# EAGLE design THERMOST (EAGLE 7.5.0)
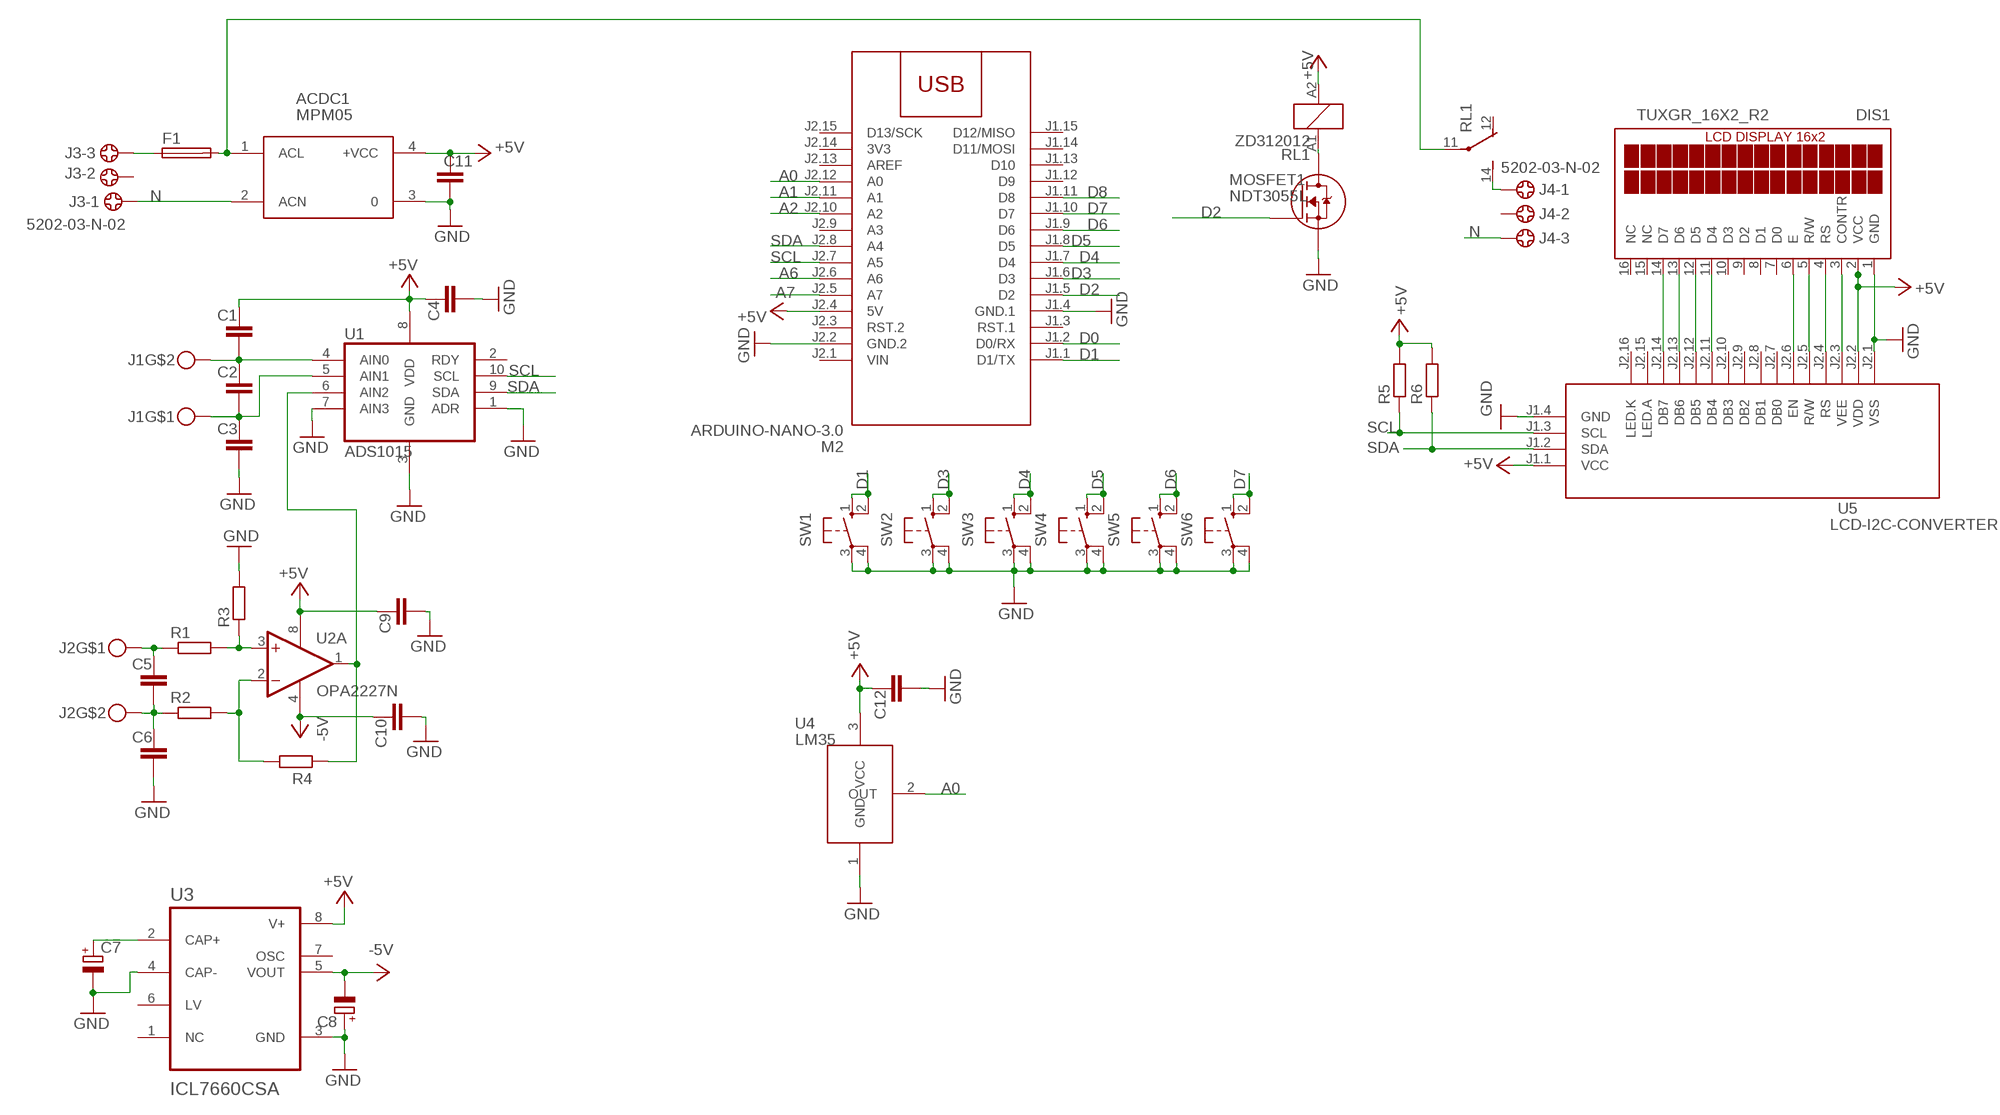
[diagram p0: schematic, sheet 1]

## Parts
ACDC1  MPM05  [MPM05]
C1  C-EUC1206  [C1206]
C2  C-EUC1206  [C1206]
C3  C-EUC1206  [C1206]
C4  C-EUC1206  [C1206]
C5  C-EUC1206  [C1206]
C6  C-EUC1206  [C1206]
C7  CPOL-EUSMCB  [SMC_B]
C8  CPOL-EUSMCB  [SMC_B]
C9  C-EUC1206  [C1206]
C10  C-EUC1206  [C1206]
C11  C-EUC1206  [C1206]
C12  C-EUC1206  [C1206]
DIS1  TUXGR_16X2_R2  [TUXGR_16X2_R2]
F1  FUSEBLANK_5X20MM  [FUSE_HOLDER_5X20MM]
J1  MKDSN1,5-2-5,08  [MKDSN1,5-2-5,08]
J2  MKDSN1,5-2-5,08  [MKDSN1,5-2-5,08]
J3  5202-03-N-02  [5202-03-N-02]
J4  5202-03-N-02  [5202-03-N-02]
M2  ARDUINO-NANO-3.0  [ARDUINO-NANO-3.0]
MOSFET1  NDT3055L  [SOT223-4]
R1  R-EU_R1206  [R1206]
R2  R-EU_R1206  [R1206]
R3  R-EU_R1206  [R1206]
R4  R-EU_R1206  [R1206]
R5  R-EU_R1206  [R1206]
R6  R-EU_R1206  [R1206]
RL1  ZD312012  [ZD1]
SW1  40-XX  [B3F-40XX]
SW2  40-XX  [B3F-40XX]
SW3  40-XX  [B3F-40XX]
SW4  40-XX  [B3F-40XX]
SW5  40-XX  [B3F-40XX]
SW6  40-XX  [B3F-40XX]
U1  ADS1015  [ADS1015]
U2  OPA2227N  [DIL08]
U3  ICL7660CSA  [SOIC127P600X175-8N]
U4  LM35  [TO92]
U5  LCD-I2C-CONVERTER  [LCD-I2C-CONVERTER]

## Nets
+5V: ACDC1.4(+VCC) C1.1 C4.1 C9.1 C11.1 C12.1 DIS1.2(VCC) M2.J2.4(5V) R5.2 R6.2 RL1.A2 U1.8(VDD) U2.8(P:V+) U3.8(V+) U4.3(VCC) U5.J1.1(VCC) U5.J2.2(VDD)
-5V: C8.- C10.1 U2.4(P:V-) U3.5(VOUT)
A0: M2.J2.12(A0) U4.2(OUT)
A1: M2.J2.11(A1)
A2: M2.J2.10(A2)
A6: M2.J2.6(A6)
A7: M2.J2.5(A7)
D0: M2.J1.2(D0/RX)
D1: M2.J1.1(D1/TX) SW1.1(S) SW1.2(S1)
D2: M2.J1.5(D2) MOSFET1.1(G)
D3: M2.J1.6(D3) SW2.1(S) SW2.2(S1)
D4: M2.J1.7(D4) SW3.1(S) SW3.2(S1)
D5: M2.J1.8(D5) SW4.1(S) SW4.2(S1)
D6: M2.J1.9(D6) SW5.1(S) SW5.2(S1)
D7: M2.J1.10(D7) SW6.1(S) SW6.2(S1)
D8: M2.J1.11(D8)
GND: ACDC1.3 C3.2 C4.2 C6.2 C7.- C8.+ C9.2 C10.2 C11.2 C12.2 DIS1.1(GND) M2.J1.4(GND.1) M2.J2.2(GND.2) MOSFET1.3(S) R3.2 SW1.3(P) SW1.4(P1) SW2.3(P) SW2.4(P1) SW3.3(P) SW3.4(P1) SW4.3(P) SW4.4(P1) SW5.3(P) SW5.4(P1) SW6.3(P) SW6.4(P1) U1.1(ADR) U1.3(GND) U1.7(AIN3) U3.3(GND) U3.4(CAP-) U4.1(GND) U5.J1.4(GND) U5.J2.1(VSS)
N: ACDC1.2(ACN) J3.1 J4.3
N$1: DIS1.14(D7) U5.J2.14(DB7)
N$2: DIS1.13(D6) U5.J2.13(DB6)
N$3: DIS1.12(D5) U5.J2.12(DB5)
N$4: DIS1.11(D4) U5.J2.11(DB4)
N$5: DIS1.6(E) U5.J2.6(EN)
N$6: DIS1.5(R/W) U5.J2.5(R/W)
N$7: DIS1.4(RS) U5.J2.4(RS)
N$8: C1.2 C2.1 J1.2 U1.4(AIN0)
N$9: R1.2 R3.1 U2.3(A:+IN)
N$10: DIS1.3(CONTR) U5.J2.3(VEE)
N$11: C2.2 C3.1 J1.1 U1.5(AIN1)
N$12: R2.2 R4.1 U2.2(A:-IN)
N$13: R4.2 U1.6(AIN2) U2.1(A:OUT)
N$14: C5.1 J2.1 R1.1
N$15: C5.2 C6.1 J2.2 R2.1
N$16: C7.+ U3.2(CAP+)
N$17: MOSFET1.2(D) MOSFET1.4(D) RL1.A1
N$18: J4.1 RL1.14(2:S)
N$19: F1.1 J3.3
N$21: ACDC1.1(ACL) F1.2 RL1.11(2:P)
SCL: M2.J2.7(A5) R5.1 U1.10(SCL) U5.J1.3(SCL)
SDA: M2.J2.8(A4) R6.1 U1.9(SDA) U5.J1.2(SDA)
Unconnected: DIS1.7(D0) DIS1.8(D1) DIS1.9(D2) DIS1.10(D3) DIS1.15(NC) DIS1.16(NC) J3.2 J4.2 M2.J1.3(RST.1) M2.J1.12(D9) M2.J1.13(D10) M2.J1.14(D11/MOSI) M2.J1.15(D12/MISO) M2.J2.3(RST.2) M2.J2.9(A3) M2.J2.13(AREF) M2.J2.15(D13/SCK) RL1.12(2:O) U1.2(RDY) U2.5(B:+IN) U2.6(B:-IN) U2.7(B:OUT) U3.1(NC) U3.6(LV) U3.7(OSC) U5.J2.7(DB0) U5.J2.8(DB1) U5.J2.9(DB2) U5.J2.10(DB3) U5.J2.15(LED.A) U5.J2.16(LED.K)

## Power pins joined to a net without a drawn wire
3V3: M2.J2.14(3V3)
VIN: M2.J2.1(VIN)

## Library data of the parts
ACDC1 = acdc:MPM05: AC DC Converter 5W
C1-C6 C9-C12 = rcl:C-EU: CAPACITOR, European symbol
C7 C8 = rcl:CPOL-EU: POLARIZED CAPACITOR, European symbol
DIS1 = display-lcd:TUXGR_16X2_R2: Tuxgraphics LCD display 16x2 characters reflective, without background light Source: tuxgr_12x2_r2.pdf; OC_FARNELL: unknown; OC_NEWARK: unknown
F1 = fuse:FUSE: Fuse; OC_FARNELL: unknown; OC_NEWARK: unknown
J1 J2 = con-phoenix-508:MKDSN1,5-2-5,08
J3 J4 = con-ebyelectro:5202-03-N-02: Barrier Blocks Sreies 5202 Source: http://www.ebyelectro.com/PDF/5202-XX-N-02.pdf; OC_FARNELL: unknown; OC_NEWARK: unknown
M2 = diy-modules:ARDUINO-NANO-3.0: Arduino Nano 3.0 and compatible devices More details available here: https://www.arduino.cc/en/Main/ArduinoBoardNano Click here to find device on ebay.com
MOSFET1 = NDT3055L:NDT3055L: Trans MOSFET N-CH 60V 4A 4-Pin(3+Tab) SOT-223 Trans MOSFET N-CH 60V 4A 4-Pin(3+Tab) SOT-223 Check availability; AVAILABILITY: In Stock; CHECK_PRICES: https://www.snapeda.com/parts/NDT3055L/Onsemi/view-part/?ref=eda; DESCRIPTION: Trans MOSFET N-CH 60V 4A 4-Pin(3+Tab) SOT-223 Trans MOSFET N-CH 60V 4A 4-Pin(3+Tab) SOT-223; MF: ON; MP: NDT3055L; PACKAGE: SOT-223-4 Fairchild Semiconductor; PRICE: None; SNAPEDA_LINK: https://www.snapeda.com/parts/NDT3055L/Onsemi/view-part/?ref=snap
R1-R6 = rcl:R-EU_: RESISTOR, European symbol
RL1 = relay:ZD?1*: Power Relay SCHRACK 1 pole 30 A Source: http://www.schrack.com/.. 5848.pdf; OC_FARNELL: unknown; OC_NEWARK: unknown
SW1-SW6 = switch-omron:40-XX: OMRON SWITCH; MF: OMRON COMPONENTS USA; MPN: B3F-4000; OC_FARNELL: 176434; OC_NEWARK: 36K3105
U1 = burr-brown:ADS1015: 12BIT I2C DAC
U2 = linear:OPA222*: High Precision, Low Noise OPERATIONAL AMPLIFIERS Source: http://focus.ti.com/lit/ds/symlink/opa227.pdf
U3 = ICL7660CSA:ICL7660CSA: Check availability; AVAILABILITY: In Stock; CHECK_PRICES: https://www.snapeda.com/parts/ICL7660CSA/Analog+Devices/view-part/?ref=eda; DESCRIPTION: Charge Pump Switching Regulator IC Positive or Negative Fixed -Vin, nVin, Vin/2 1 Output 20mA 8-SOIC (0.154, 3.90mm Width); MF: Analog Devices; MP: ICL7660CSA; PACKAGE: SOIC-8 Maxim; PRICE: None; SNAPEDA_LINK: https://www.snapeda.com/parts/ICL7660CSA/Analog+Devices/view-part/?ref=snap
U4 = transistor-neu-to92:LM35: Precision Centigrade Temperature Sensor (-55C to 150C)
U5 = diy-modules:LCD-I2C-CONVERTER: I2C Bus to 4-Bit Parallel LCD Interface with LED backlight driver

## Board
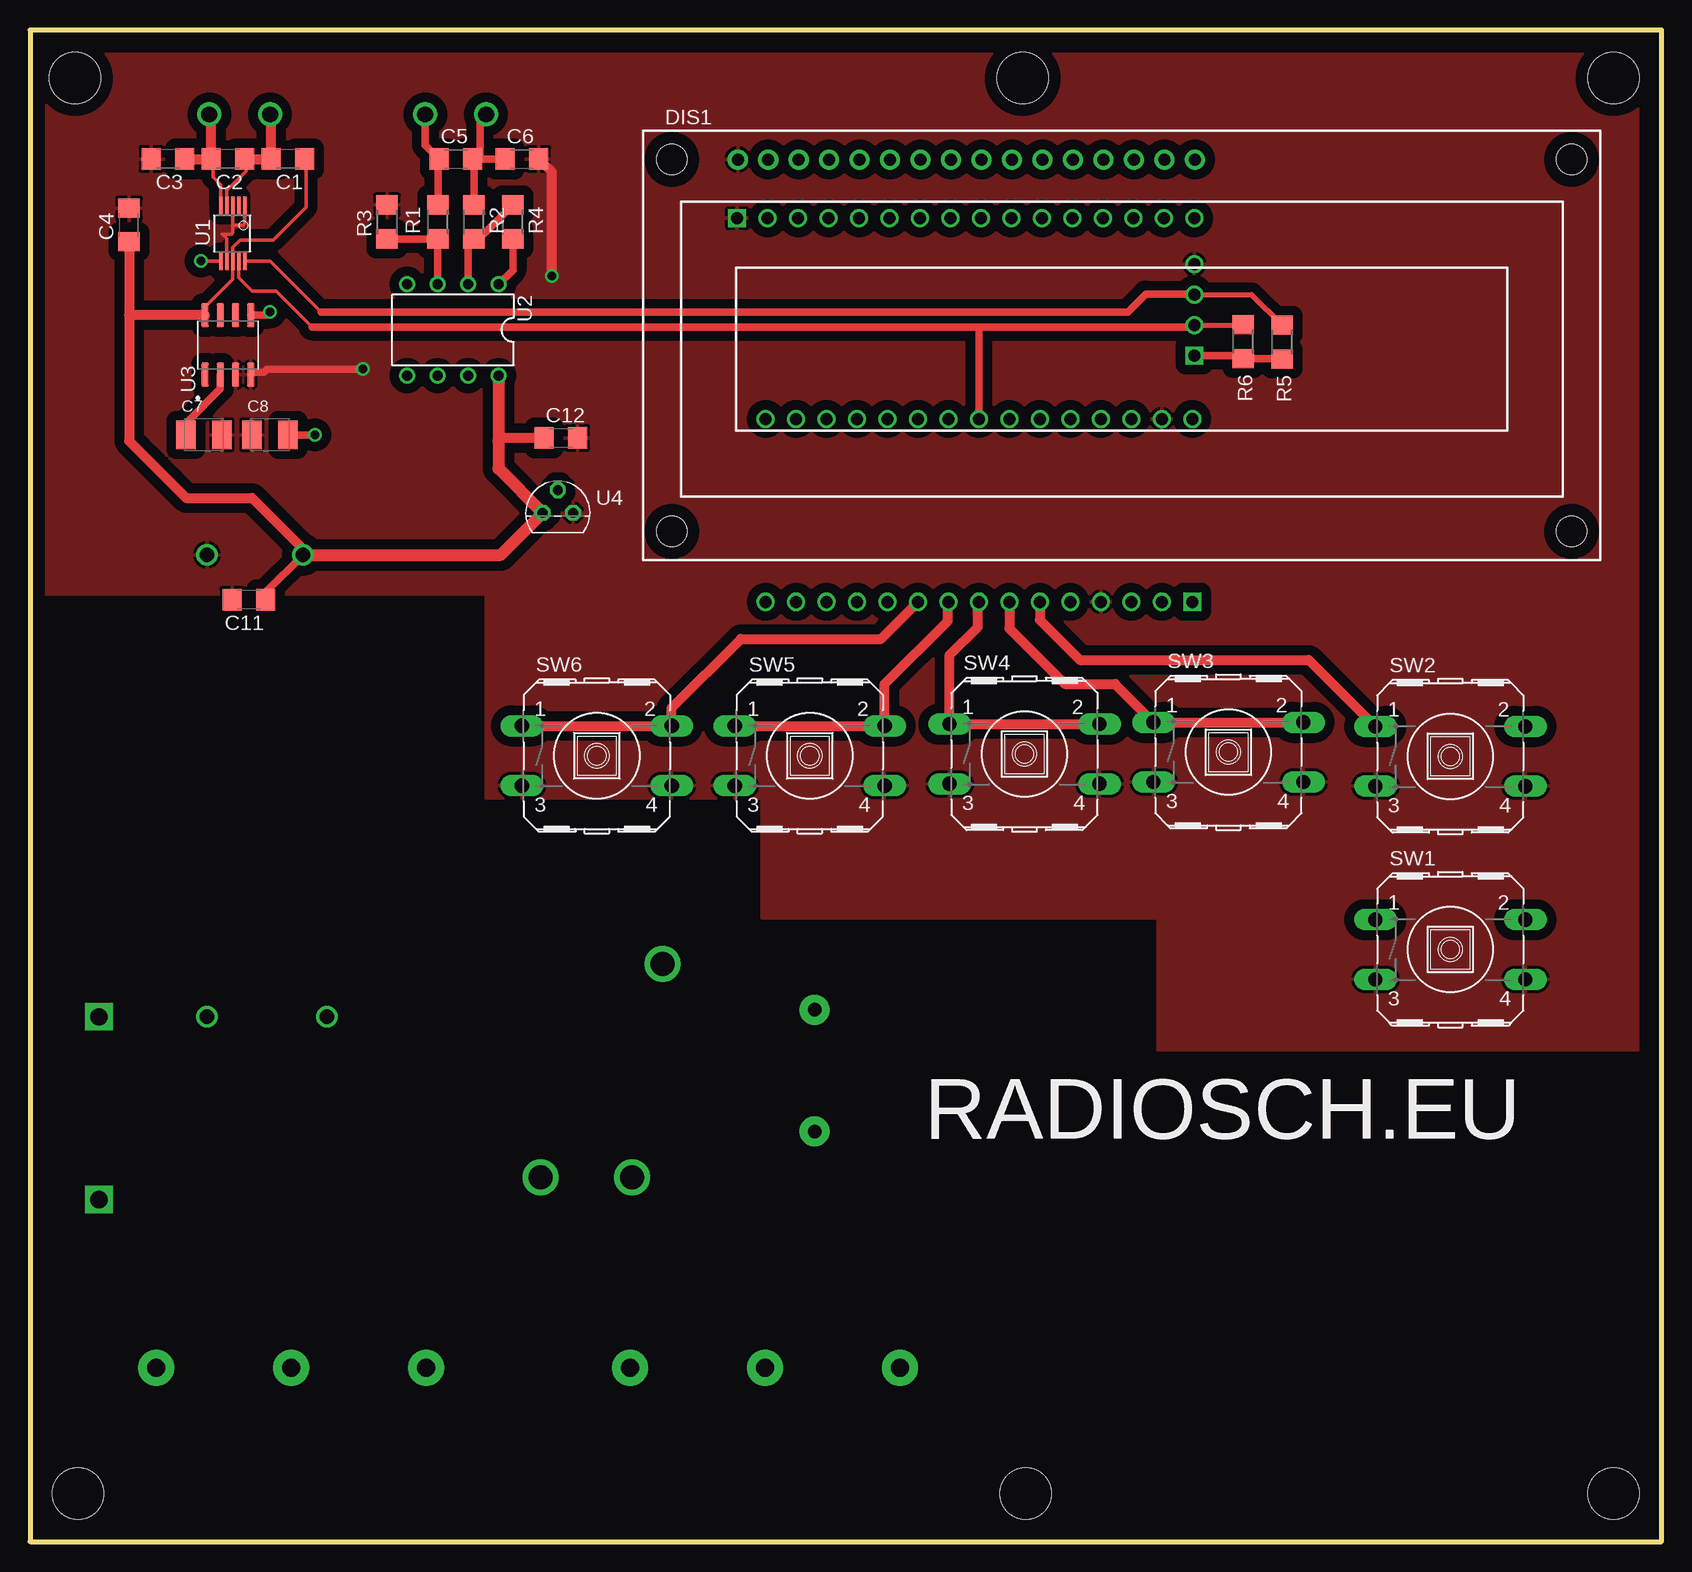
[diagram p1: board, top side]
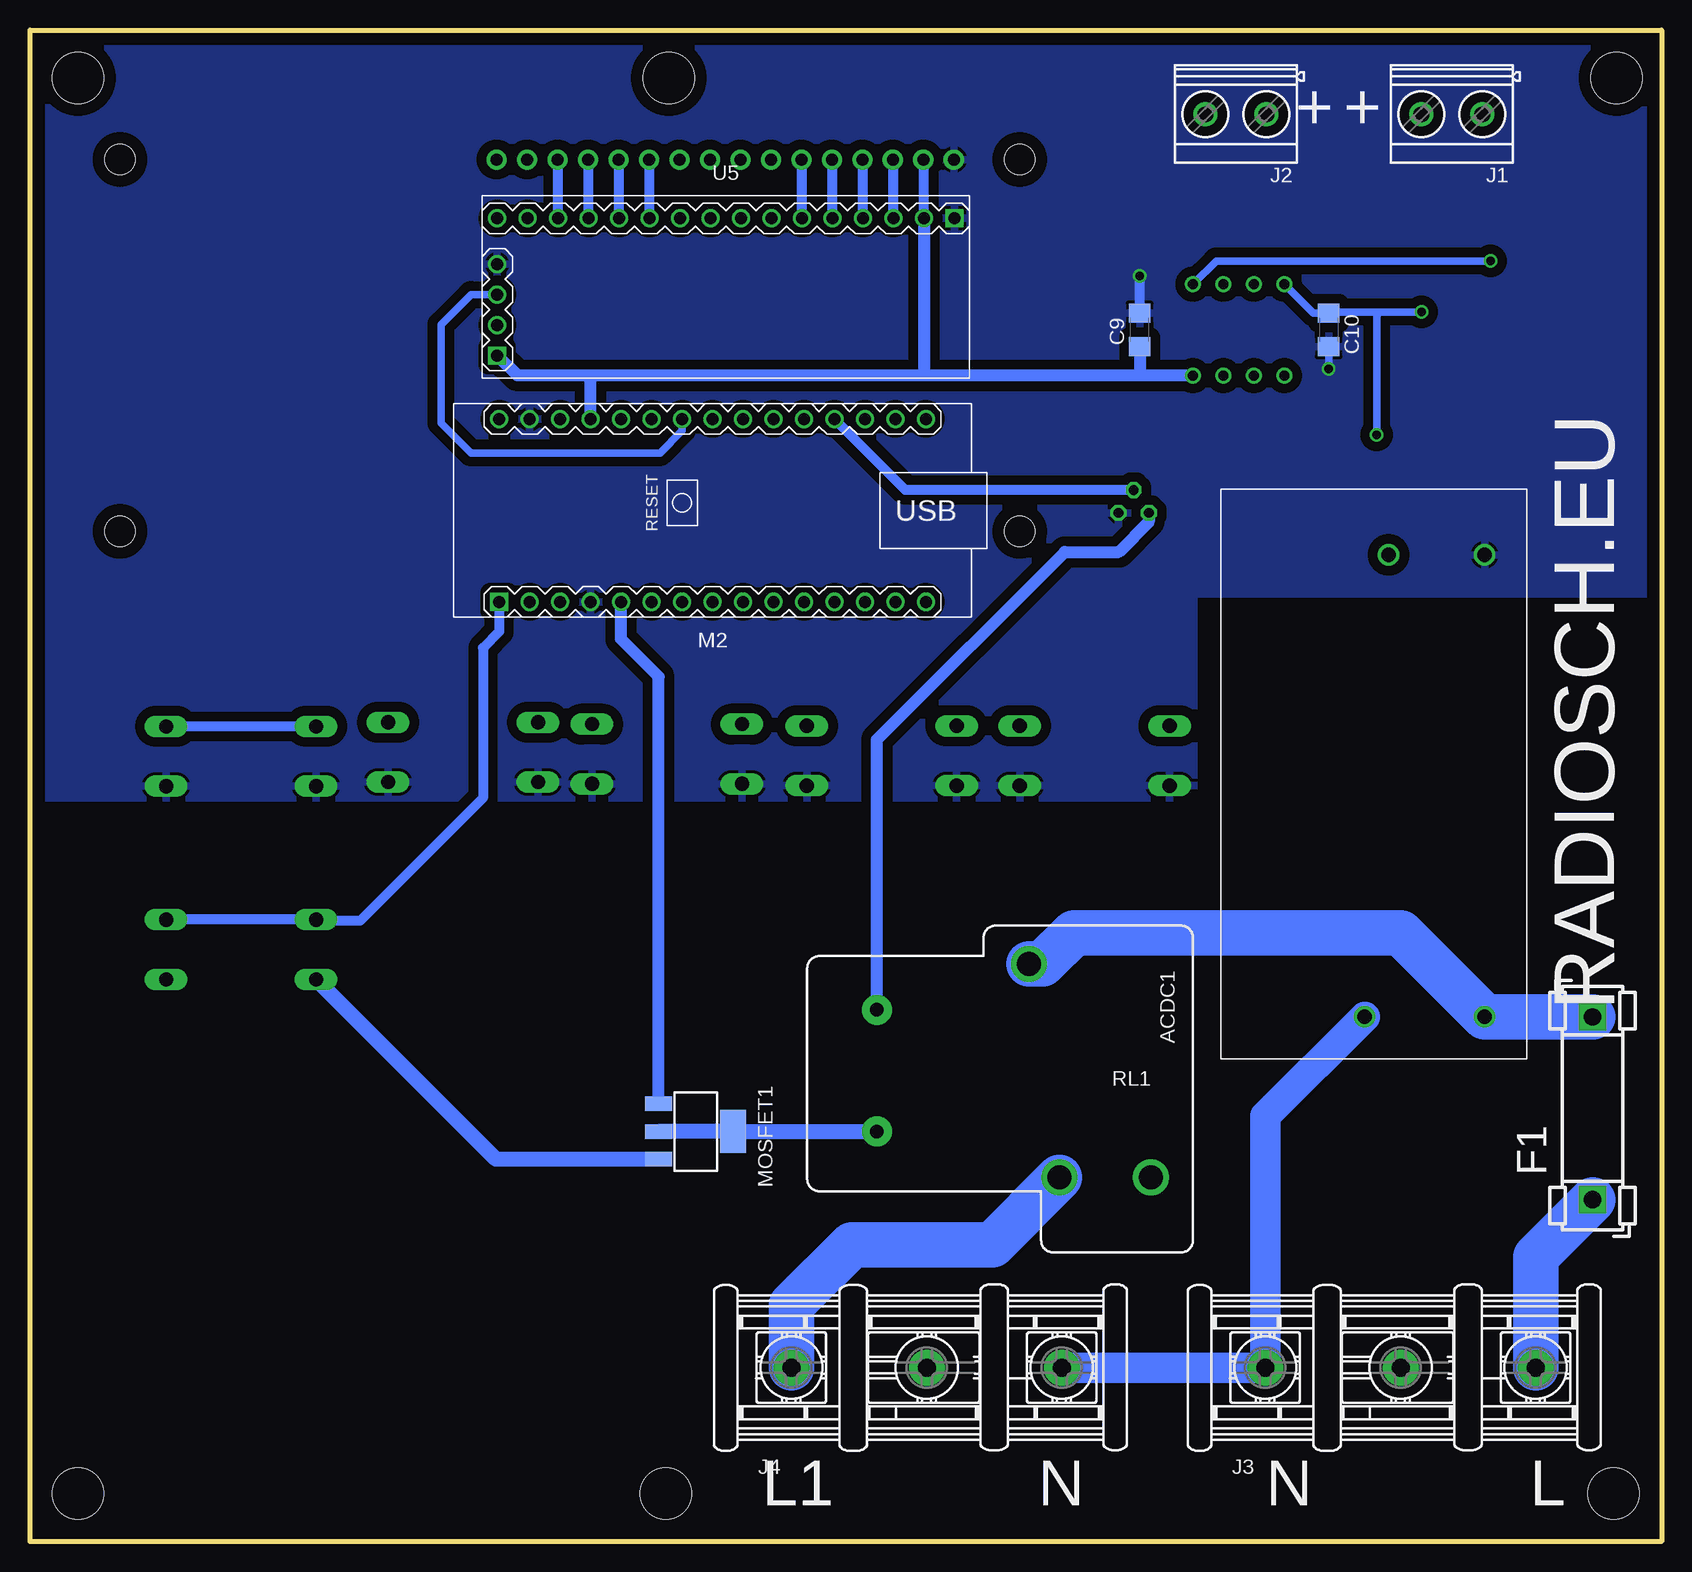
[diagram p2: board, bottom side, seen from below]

Size 136 x 126 mm. Coordinates in mm from the lower left corner, seen from the top.
Outline: 0,0 136,0 136,126 0,126 0,0
Copper layers (1*16): Top 0.035mm / dielectric 1.5mm / Bottom 0.035mm
Design rules "default *": minimum track width 10mil, minimum drill 24mil, track to track 4mil, track to pad 6mil, pad to pad 4mil, via to via 8mil, smd to smd 8mil, copper to edge 40mil, drill to drill 8mil, minimum pad ring 10mil, minimum via ring 8mil, stop-mask expansion 4mil, vias tented up to drill 0mil, thermal gap 10mil
Holes 4.3 mm at 3.75,122 4,4 132,4 132,122 83,4 82.75,122

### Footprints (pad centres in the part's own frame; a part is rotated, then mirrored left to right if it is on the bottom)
MPM05 = drill 1.2: 1 3.5,-22; 2 3.5,-12; 3 42,-22; 4 42,-14
C1206 = smd 1.6 x 1.8: 1 -1.4,0; 2 1.4,0
SMC_B = smd 1.6 x 2.4: + -1.5,0; - 1.5,0
TUXGR_16X2_R2 = drill 1 pad 1.676: 1 -32,15.5; 2 -29.46,15.5; 3 -26.92,15.5; 4 -24.38,15.5; 5 -21.84,15.5; 6 -19.3,15.5; 7 -16.76,15.5; 8 -14.22,15.5; 9 -11.68,15.5; 10 -9.14,15.5; 11 -6.6,15.5; 12 -4.06,15.5; 13 -1.52,15.5; 14 1.02,15.5; 15 3.56,15.5; 16 6.1,15.5 | hole 2.5: -37.5,-15.5; 37.5,-15.5; -37.5,15.5; 37.5,15.5
FUSE_HOLDER_5X20MM = drill 1.422 pad 2.286 square: 1 0,0; 2 15.24,0
MKDSN1,5-2-5,08 = drill 1.3 pad 2: 1 -2.561,0.025; 2 2.519,0.025
5202-03-N-02 = drill 1.5 pad 3: 1 -9.29,0; 2 2,0; 3 13.25,0
ARDUINO-NANO-3.0 = drill 1 square: J1.1 17.78,7.62 | drill 1: J1.2 15.24,7.62; J1.3 12.7,7.62; J1.4 10.16,7.62; J1.5 7.62,7.62; J1.6 5.08,7.62; J1.7 2.54,7.62; J1.8 0,7.62; J1.9 -2.54,7.62; J1.10 -5.08,7.62; J1.11 -7.62,7.62; J1.12 -10.16,7.62; J1.13 -12.7,7.62; J1.14 -15.24,7.62; J1.15 -17.78,7.62; J2.1 17.78,-7.62; J2.2 15.24,-7.62; J2.3 12.7,-7.62; J2.4 10.16,-7.62; J2.5 7.62,-7.62; J2.6 5.08,-7.62; J2.7 2.54,-7.62; J2.8 0,-7.62; J2.9 -2.54,-7.62; J2.10 -5.08,-7.62; J2.11 -7.62,-7.62; J2.12 -10.16,-7.62; J2.13 -12.7,-7.62; J2.14 -15.24,-7.62; J2.15 -17.78,-7.62
SOT223-4 = smd 1.219 x 2.235: 1 -2.24,-3.091; 2 0.071,-3.091; 3 2.383,-3.091 | smd 3.6 x 2.2: 4 0.071,3.107
R1206 = smd 1.6 x 1.803: 1 -1.422,0; 2 1.422,0
ZD1 = drill 2 pad 2.5: 11 -2.54,-8.88; 12 -12.7,8.88; 14 -5.08,8.88 | drill 1.1 pad 2.5: A1 10.16,5.08; A2 10.16,-5.08
B3F-40XX = drill 1.194 long: 1 -6.248,2.489; 2 6.248,2.489; 3 -6.248,-2.489; 4 6.248,-2.489
ADS1015 = smd 0.3 x 1.5: 1 -1.905,-2.616; 2 -1.405,-2.616; 3 -0.905,-2.616; 4 -0.405,-2.616; 5 0.095,-2.616; 6 0.095,1.984; 7 -0.405,1.984; 8 -0.905,1.984; 9 -1.405,1.984; 10 -1.905,1.984
DIL08 = drill 0.813 pad 1.27: 1 -3.81,-3.81; 2 -1.27,-3.81; 3 1.27,-3.81; 4 3.81,-3.81; 5 3.81,3.81; 6 1.27,3.81; 7 -1.27,3.81; 8 -3.81,3.81
SOIC127P600X175-8N = smd 1.97 x 0.59: 1 -2.475,1.905; 2 -2.475,0.635; 3 -2.475,-0.635; 4 -2.475,-1.905; 5 2.475,-1.905; 6 2.475,-0.635; 7 2.475,0.635; 8 2.475,1.905
TO92 = drill 0.813 octagon: 1 1.27,0; 2 0,1.905; 3 -1.27,0
LCD-I2C-CONVERTER = drill 1 square: J1.1 -19.05,-5.08; J2.1 19.05,6.35 | drill 1: J1.2 -19.05,-2.54; J1.3 -19.05,0; J1.4 -19.05,2.54; J2.2 16.51,6.35; J2.3 13.97,6.35; J2.4 11.43,6.35; J2.5 8.89,6.35; J2.6 6.35,6.35; J2.7 3.81,6.35; J2.8 1.27,6.35; J2.9 -1.27,6.35; J2.10 -3.81,6.35; J2.11 -6.35,6.35; J2.12 -8.89,6.35; J2.13 -11.43,6.35; J2.14 -13.97,6.35; J2.15 -16.51,6.35; J2.16 -19.05,6.35

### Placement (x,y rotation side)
ACDC1  36.75,40.25 90 bottom
C1  21.5,115.25 180 top
C2  16.5,115.25 180 top
C3  11.5,115.25 180 top
C4  8.25,109.75 90 top
C5  35.5,115.25 0 top
C6  41,115.25 0 top
C7  14.5,92.25 0 top
C8  20,92.25 0 top
C9  43.5,101 90 bottom
C10  27.75,101 270 bottom
C11  18.25,78.5 180 top
C12  44.25,92 0 top
DIS1  91,99.7 0 top
F1  5.75,28.5 90 bottom
J1  17.5,119 180 bottom
J2  35.5,119 180 bottom
J3  23.75,14.5 0 bottom
J4  63.25,14.5 0 bottom
M2  79.1,85.95 180 bottom
MOSFET1  80.5,34.25 270 bottom
R1  34,110 270 top
R2  37,110 270 top
R3  29.75,110 90 top
R4  40.25,110 270 top
R5  104.38,99.97 270 top
R6  101.12,100.03 270 top
RL1  55.25,39.25 180 bottom
SW1  118.4,49.35 0 top
SW2  118.4,65.45 0 top
SW3  99.9,65.8 0 top
SW4  82.9,65.65 0 top
SW5  65,65.5 0 top
SW6  47.25,65.5 0 top
U1  16,108.72 180 top
U2  35.25,101 180 top
U3  16.5,99.75 90 top
U4  44,85.75 0 top
U5  78,103.95 0 bottom

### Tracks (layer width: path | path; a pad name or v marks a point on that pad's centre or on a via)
+5V
  Top 0.305: U3.8 14.59,102.94 16.91,105.25 U1.8 16.91,107.91 17.5,108.5 20.25,108.5 23,111.25 23,115.15 C1.1
  Top 0.61: U5.J1.1 100.86,98.87 R6.2 104.33,98.6 R5.2 | C11.1 19.65,79.15 ACDC1.4
  Top 0.813: C4.1 8.25,102.25 | 8.25,102.25 8.25,91.75 13,87 18.5,87 23.25,82.25 | U3.8 8.27,102.22 8.25,102.25 | C12.1 39.31,92 39.06,91.75
  Top 1.016: ACDC1.4 23.25,82.25 39.23,82.25 U4.3 39.06,89.42 39.06,91.75 U2.8
  Bottom 0.813: U5.J2.2 61.49,115.15 DIS1.2
  Bottom 1.016: U2.8 43.75,97.19 | 43.75,97.19 61.25,97.19 | 61.25,97.19 89,97.19 | 89,97.19 95.37,97.19 U5.J1.1 | M2.J2.4 89.26,96.93 89,97.19 | C9.1 43.5,97.44 43.75,97.19 | U5.J2.2 61.49,97.43 61.25,97.19 | U4.3 42.73,85.02 45.25,82.5 49.75,82.5 65.41,66.84 RL1.A2
-5V  (via drill 0.7)
  Top 0.61: C8.- v23.75,92.25 | U3.5 19.73,102.22 v20,102.5
  Bottom 0.61: U2.4 29.03,102.4 C10.1 27.65,102.5 23.5,102.5 | v23.75,92.25 23.75,102.25 23.5,102.5 | v20,102.5 23.5,102.5
A0
  Bottom 0.813: U4.2 63.02,87.66 M2.J2.12
D1
  Bottom 0.813: M2.J1.1 96.88,75.87 98.25,74.5 98.25,62 108.5,51.75 112.06,51.75 SW1.1 SW1.2
D2
  Bottom 1.016: M2.J1.5 86.75,78.3 86.75,75.25 83.59,72.09 MOSFET1.1
D3
  Top 0.813: M2.J1.6 84.18,76.82 87.5,73.5 106.59,73.5 SW2.1
  Bottom 0.813: SW2.1 SW2.2
D4
  Top 0.813: M2.J1.7 81.64,76.11 86.25,71.5 90.44,71.5 SW3.1 SW3.2
D5
  Top 0.813: M2.J1.8 79,78.23 79,76.25 76.65,73.9 SW4.1 SW4.2
D6
  Top 0.813: SW5.2 71.25,68.5 | 71.25,68.5 71.25,71.5 76.5,76.75 76.5,78.27 M2.J1.9 | SW5.1 70.74,67.99 71.25,68.5
D7
  Top 0.813: M2.J1.10 70.94,75.25 59.25,75.25 53.5,69.5 SW6.2 SW6.1
GND  (via drill 0.7)
  Top 0.305: U1.3 16.91,109.75 | 16.91,109.75 16.91,109.09 16.81,109 16,109 16.41,108.59 U1.7 | U1.1 17.91,109.91 17.75,109.75 16.91,109.75
  Top 0.61: v27.75,97.75 19.75,97.75 19.5,97.5 18.63,97.5 U3.4
  Top 0.813: v43.5,105.5 43.5,114.15 C6.2
  Bottom 0.61: C10.2 v27.75,97.75
  Bottom 0.813: C9.2 v43.5,105.5
  Bottom 1.27: MOSFET1.3 97.16,31.87 SW1.3
  pour Top (isolate 0.813): 0,124 134,124 134,41 94,41 94,52 61,52 61,61 61,62 38,62 38,79 0,79
  pour Bottom (isolate 0.813): 1,79 39,79 39,62 135,62 135,125 1,125
N
  Bottom 2.54: ACDC1.2 33.04,35.46 J3.1 J4.3
N$1
  Bottom 0.813: U5.J2.14 91.97,115.15 DIS1.14
N$2
  Bottom 0.813: U5.J2.13 89.43,115.15 DIS1.13
N$3
  Bottom 0.813: U5.J2.12 86.89,115.15 DIS1.12
N$4
  Bottom 0.813: U5.J2.11 84.35,115.15 DIS1.11
N$5
  Bottom 0.813: U5.J2.6 71.65,115.15 DIS1.6
N$6
  Bottom 0.813: U5.J2.5 69.11,115.15 DIS1.5
N$7
  Bottom 0.813: U5.J2.4 66.57,115.15 DIS1.4
N$8
  Top 0.305: U1.4 16.41,112.66 18,114.25 18,115.15 C2.1
  Top 0.813: C2.1 C1.2 20.1,118.89 J1.2
N$9
  Top 0.61: U2.3 33.98,108.56 R1.2 R3.1
N$10
  Bottom 0.813: U5.J2.3 64.03,115.15 DIS1.3
N$11
  Top 0.305: U1.5 15.91,113.09 15.25,113.75 15.25,115.1 C2.2
  Top 0.813: C3.1 C2.2 15.1,118.81 J1.1
N$12
  Top 0.61: U2.2 36.52,108.1 R2.2 37.41,108.58 R4.1
N$13  (via drill 0.7)
  Top 0.305: U1.6 v14.26,106.74 v14.25,106.75
  Top 0.61: R4.2 40.25,106 U2.1
  Bottom 0.61: v14.25,106.75 37.12,106.75 U2.1
N$14
  Top 0.61: R1.1 34,115.15 C5.1 32.94,116.41 J2.1
N$15
  Top 0.61: R2.1 37,114.75 37.5,115.25 | C6.1 37.5,115.25 | 37.5,115.25 C5.2 | 37.5,115.25 37.5,118.46 J2.2
N$16
  Top 0.61: U3.2 15.86,96.11 13.25,93.5 13.25,92.5 C7.+
N$17
  Bottom 1.27: MOSFET1.2 MOSFET1.4 RL1.A1
N$18
  Bottom 3.81: J4.1 72.54,19.71 67.5,24.75 55.79,24.75 RL1.14
N$19
  Bottom 3.81: J3.3 10.5,23.75 F1.1
N$21
  Bottom 3.81: F1.2 ACDC1.1 21.75,50.75 49,50.75 51.62,48.13 RL1.11
SCL
  Top 0.305: U1.10 20.01,106.74 24.25,102.5
  Top 0.406: U5.J1.3 101.82,103.95 R5.1
  Top 0.61: 24.25,102.5 91.5,102.5 93,104 97,104 U5.J1.3
  Bottom 0.61: M2.J2.7 81.64,92.61 83.5,90.75 99.25,90.75 101.75,93.25 101.75,101.45 99.25,103.95 U5.J1.3
SDA
  Top 0.305: U1.9 17.41,105.34 18.5,104.25 20.5,104.25 23.5,101.25
  Top 0.406: U5.J1.2 101.09,101.41 R6.1
  Top 0.61: 23.5,101.25 79.25,101.25 | 79.25,101.25 96.89,101.25 U5.J1.2 | M2.J2.8 79.1,101.1 79.25,101.25

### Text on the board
tPlace: RADIOSCH.EU
bPlace: + | + | RADIOSCH.EU | L | N | N | L1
